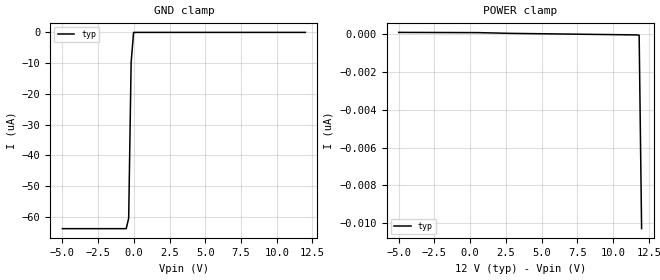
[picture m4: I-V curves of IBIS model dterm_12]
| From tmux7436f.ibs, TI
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| dterm_12
[Model]   dterm_12
Model_type   Terminator
|   typ   min   max
C_comp   4.014581e-12   NA   NA
[Voltage Range]   12   NA   NA
[Temperature Range]   27   NA   NA
[Power Clamp Reference]   12   NA   NA
[GND Clamp Reference]   0   NA   NA
[GND Clamp]
|   Voltage   I(typ)   I(min)   I(max)
-5V       -63.89uA   NA         NA
-535.4mV  -63.88uA   NA         NA
-363.6mV  -60.5uA    NA         NA
-191.9mV  -9.798uA   NA         NA
-20.2mV   -22.4nA    NA         NA
12V       100pA      NA         NA
[POWER Clamp]
|   Voltage   I(typ)   I(min)   I(max)
-5V       110.3pA    NA         NA
494.9mV   98.94pA    NA         NA
11.83V    -38.63pA   NA         NA
12V       -10.29nA   NA         NA
